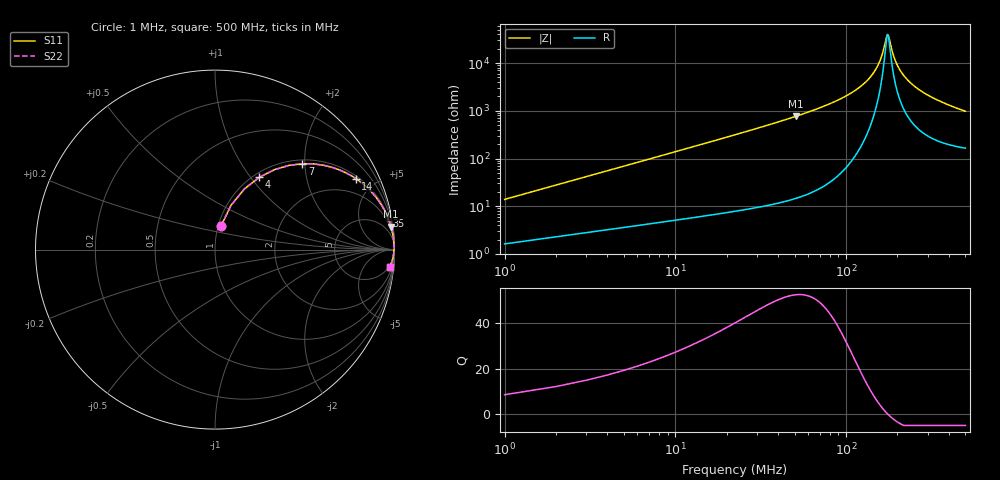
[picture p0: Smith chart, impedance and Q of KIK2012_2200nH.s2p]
!version-2
!date-01.2022
!Series
# MHz S RI R 50
!Freq ReS11 ImS11 ReS21 ImS21 ReS12 ImS12 ReS22 ImS22
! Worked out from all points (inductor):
!   500 points, 1 MHz to 500 MHz, reference 50 ohm
!   read as one part in series: L = 2.2 uH near 3 MHz
!   highest Q = 52.5 at 51 MHz (marker M1), where L = 2.4 uH
!   self-resonance near 175 MHz
!   S11 on the Smith chart (normalised r, x): 1 MHz: 1.03, +0.28; 4 MHz: 1.06, +1.11; 7 MHz: 1.09, +1.94; 14 MHz: 1.12, +3.90; 35 MHz: 1, +10; 500 MHz: 4, -19
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1  0.0339 0.1314  0.9661 -0.1314  0.9661 -0.1314  0.0339 0.1314
4  0.2474 0.4034  0.7526 -0.4034  0.7526 -0.4034  0.2474 0.4034
7  0.4855 0.4783  0.5145 -0.4783  0.5145 -0.4783  0.4855 0.4783
10  0.6529 0.458  0.3471 -0.458  0.3471 -0.458  0.6529 0.458
14  0.7843 0.396  0.2157 -0.396  0.2157 -0.396  0.7843 0.396
22  0.8994 0.2886  0.1006 -0.2886  0.1006 -0.2886  0.8994 0.2886
35  0.9585 0.1894  0.0415 -0.1894  0.0415 -0.1894  0.9585 0.1894
51  0.9811 0.127  0.0189 -0.127  0.0189 -0.127  0.9811 0.127
85  0.9942 0.0646  0.00577 -0.0646  0.00577 -0.0646  0.9942 0.0646
119  0.9973 0.0326  0.0027 -0.0326  0.0027 -0.0326  0.9973 0.0326
141  0.9978 0.0181  0.00221 -0.0181  0.00221 -0.0181  0.9978 0.0181
157  0.9978 0.00912  0.00223 -0.00912  0.00223 -0.00912  0.9978 0.00912
168  0.9976 0.00356  0.00237 -0.00356  0.00237 -0.00356  0.9976 0.00356
173  0.9975 0.00115  0.00246 -0.00115  0.00246 -0.00115  0.9975 0.00115
176  0.9975 -0.000253  0.00252 0.000253  0.00252 0.000253  0.9975 -0.000253
190  0.9971 -0.00651  0.00288 0.00651  0.00288 0.00651  0.9971 -0.00651
203  0.9967 -0.0119  0.0033 0.0119  0.0033 0.0119  0.9967 -0.0119
223  0.9959 -0.0197  0.0041 0.0197  0.0041 0.0197  0.9959 -0.0197
251  0.9945 -0.0297  0.00547 0.0297  0.00547 0.0297  0.9945 -0.0297
334  0.9891 -0.0552  0.0109 0.0552  0.0109 0.0552  0.9891 -0.0552
417  0.982 -0.077  0.018 0.077  0.018 0.077  0.982 -0.077
500  0.9735 -0.0964  0.0265 0.0964  0.0265 0.0964  0.9735 -0.0964
